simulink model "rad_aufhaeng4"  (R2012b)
settings: Solver=ode45  StartTime=0.0  StopTime=10.0  RelTol=1e-3
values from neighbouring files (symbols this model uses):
  a1 = subplot(311), plot(t, vy-vb)    [coulomb_10.m]    (also in coulomb_11.m; coulomb_2.m = subplot(311),  plot(t, y1); coulomb_3.m = subplot(311),  plot(t, y1); coulomb_5.m = subplot(311),  plot(t, y1))
  b1 = b{1}    [rad_aufhaeng_3.m]    (also in rad_aufhaeng_4.m; unwucht_2.m = b1{:})
  b2 = b{2}    [rad_aufhaeng_3.m]    (also in rad_aufhaeng_4.m)
  dt = 0.001    [coulomb_1.m]    (also in coulomb_10.m; coulomb_11.m; coulomb_2.m; coulomb_3.m)
  Fs = 1/dt    (= 500)    [unwucht_rueckw_1.m]
  Hz = inv(s^2*M + s*C + K)*Pz    [suspension_1.m]    (also in suspension_2.m; suspension_3.m)
  nfft = 512    [diff_filter_1.m]    (also in diff_filter_2.m; feder_masse_1.m = 256; feder_masse_13.m = length(u); feder_masse_14.m = length(u))
  varianz = 1e-6    (= 1e-06)    [diff_filter_1.m]    (also in diff_filter_2.m = 1e-08; rad_aufhaeng_4.m = 2e-06; suspension_2.m = 2e-06; suspension_3.m = 2e-06)
undefined symbols (not defined in the file or in its folder): dBW, get, Hertz, sided, Two
libraries: dspsnks4 x2, dspspect3 x1, dspstat3 x1, dspmtrx3 x1

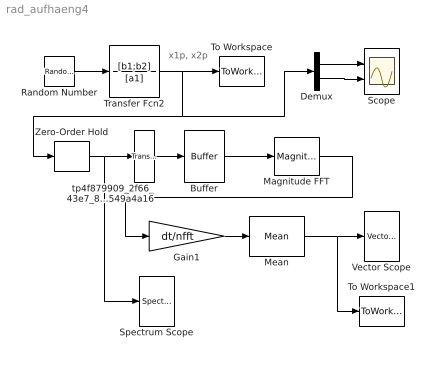
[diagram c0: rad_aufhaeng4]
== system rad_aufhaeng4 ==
  note: x1p, x2p
  Buffer : Buffer  N=nfft  V=50  TreatMby1Signals=One channel
  Demux : Demux  Outputs=2
  Gain1 : Gain  Gain=dt/nfft
  Magnitude FFT : dspspect3/Magnitude FFT  mag_or_magsq=Magnitude squared  FFTImplementation=Auto  fftLenInherit=on  fftsize=256
  Mean : dspstat3/Mean  run=on  reset_popup=None  directionMode=Each column  dimension=1  treatSBRowAsCol=on  roiEnable=off  roiType=Rectangles  roiPortion=Entire ROI  roiOutput=Individual statistics for each ROI  roiFlag=off  outputDataTypeStr=Inherit: Same as accumulator  outputLastDataTypeStr=Inherit: Same as accumulator  outputMin=[]  outputMax=[]  roundingMode=Floor  overflowMode=off
  Random Number : RandomNumber  Variance=varianz  SampleTime=dt
  Scope : Scope  NumInputPorts=2
  Spectrum Scope : dspsnks4/Spectrum Scope  ScopeProperties=on  Domain=Frequency  HorizSpan=1  UseBuffer=on  BufferSize=256  Overlap=50  TreatMby1Signals=M channels  inpFftLenInherit=off  FFTlength=128  numAvg=40  DisplayProperties=off  AxisGrid=on  Memory=off  FrameNumber=on  AxisLegend=off  AxisZoom=off  OpenScopeAtSimStart=on  OpenScopeImmediately=off  FigPos=[520 502 560 420]  AxisProperties=off  XUnits=Hertz  XRange=Two-sided ((-Fs/2...Fs/2])  XDisplay=0  InheritXIncr=off  XIncr=dt  XLabel=Samples  XLimit=User-defined  YUnits=dBW/Hertz  XMax=50  XMin=-50  YLabel=dBW/Hz  LineProperties=off  LineMarkers=|*  wintypeSpecScope=Hann  RsSpecScope=50  betaSpecScope=5  winsampSpecScope=Symmetric  XAxisParamsVer=6.9  isFrameUpgraded=on
  To Workspace : ToWorkspace  VariableName=x  SampleTime=-1  SaveFormat=Structure With Time
  To Workspace1 : ToWorkspace  VariableName=Xfft  SampleTime=-1
  Transfer Fcn2 : TransferFcn  Numerator=[b1;b2]  Denominator=[a1]
  Vector Scope : dspsnks4/Vector Scope  ScopeProperties=on  Domain=Frequency  HorizSpan=1  DisplayProperties=off  AxisGrid=on  Memory=off  FrameNumber=on  AxisLegend=off  AxisZoom=off  OpenScopeAtSimStart=on  OpenScopeImmediately=off  FigPos=get(0,'defaultfigureposition')  AxisProperties=off  XUnits=Hertz  XRange=[-Fs/2...Fs/2]  InheritXIncr=off  XIncr=dt  XLabel=Time  XLimit=Auto  XMin=0  XMax=50  XStart=0  YUnits=dB  YLabel=dBW/Hz  LineProperties=off  XAxisParamsVer=6.9
  Zero-Order Hold : ZeroOrderHold  SampleTime=dt
  tp4f879909_2f66_43e7_80cc_e430549a4a16 : dspmtrx3/Transpose  Hermitian=off  overflowFlag=off
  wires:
  Random Number/1 -> Transfer Fcn2/1
  Mean/1 -> Vector Scope/1, To Workspace1/1
  Zero-Order Hold/1 -> Spectrum Scope/1, tp4f879909_2f66_43e7_80cc_e430549a4a16/1
  Transfer Fcn2/1 -> To Workspace/1, Demux/1, Zero-Order Hold/1
  Demux/1 -> Scope/1
  Demux/2 -> Scope/2
  Magnitude FFT/1 -> Gain1/1
  Buffer/1 -> Magnitude FFT/1
  Gain1/1 -> Mean/1
  tp4f879909_2f66_43e7_80cc_e430549a4a16/1 -> Buffer/1
